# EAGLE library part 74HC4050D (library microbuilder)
6-channel level shifter 74HC4050D - 2V-6V Supply Digikey: 74HC4050D,653-ND Mouser: 771-74HC4050D-T
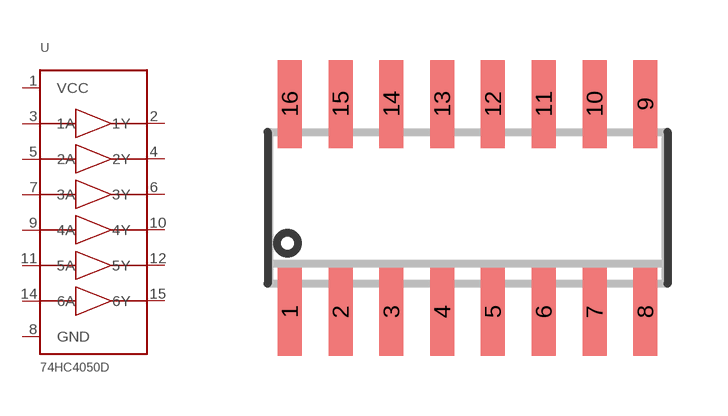
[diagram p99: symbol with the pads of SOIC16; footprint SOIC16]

Designator prefix U

## 74HC4050D  [SOIC16]
1  VCC
2  1Y
3  1A
4  2Y
5  2A
6  3Y
7  3A
8  GND
9  4A
10  4Y
11  5A
12  5Y
14  6A
15  6Y

## Footprint SOIC16 (pad centres in mm)
SMALL OUTLINE INTEGRATED CIRCUIT
smd 0.6 x 2.2: 1 -4.445,-2.6; 2 -3.175,-2.6; 3 -1.905,-2.6; 4 -0.635,-2.6; 5 0.635,-2.6; 6 1.905,-2.6; 7 3.175,-2.6; 8 4.445,-2.6; 9 4.445,2.6; 10 3.175,2.6; 11 1.905,2.6; 12 0.635,2.6; 13 -0.635,2.6; 14 -1.905,2.6; 15 -3.175,2.6; 16 -4.445,2.6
